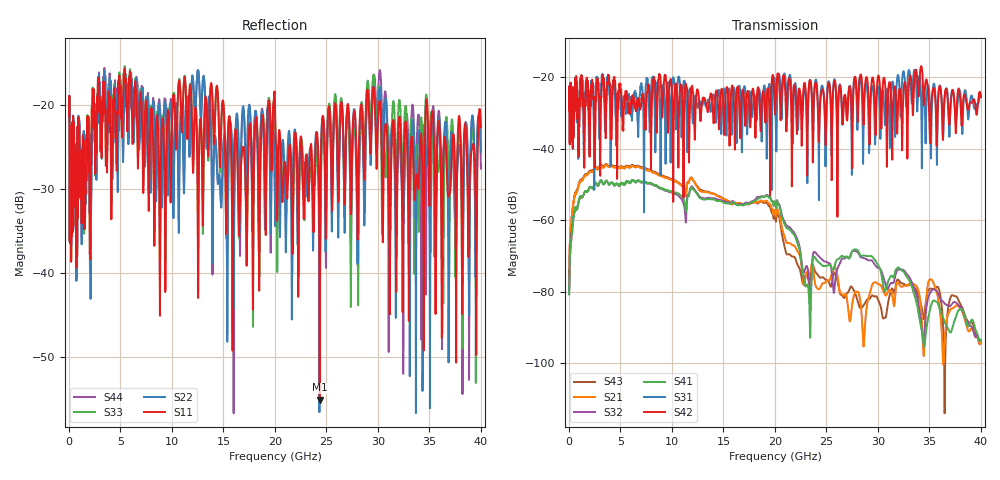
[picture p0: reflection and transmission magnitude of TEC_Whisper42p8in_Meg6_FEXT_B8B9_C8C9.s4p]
! Tyco Electronics Strada Whisper System
! FEXT_B8B9-C8C9
!! SYSTEM DESCRIPTION: Daughtercard-Connector-Backplane-Connector-Daughtercard
!! PCB DESCRIPTION: BP: 250mil, 26 lyrs, Megtron6, bottom layer route, no stub, 6-9-6mil 30" traces; DC: 150mil, 16 lyrs, Megtron6, bottom layer route, no stub, 6-9-6mil 5" traces
!! CONNECTOR DESCRIPTION: STRADA Whisper, Right Angle Receptacle to Vertical Header
!! MODEL DESCRIPTION: Tyco Electronics System 4-port S-parameter
!! MODEL STATUS: Developmental
!! MODEL GEOMETRY: Channel Model
!! MODEL FREQUENCY RANGE: DC to 40 GHz in 10 MHz frequency steps
!! MODEL EDGE RATE LIMITATION: 12.5 ps (Using conservative 0.5/Fmax rule of thumb)
!! TIME-DOMAIN TRANSFORM CAUTIONS:
!! 1.) Do not simulate transient edge rates faster than the number listed above.  Edge rates faster than this number
!!  contain significant spectral content at frequencies above the model's highest frequency.
!! 2.) Even when simulating edge rates that are slower than the number listed above, be aware that the best time
!!  resolution possible with a direct iFFT is (1 / 2Fmax).  As a result, time resolution is typically not adequate
!!  for most time-domain simulations unless tricks such as windowing are used to minimize leakage and aliasing.
!! 3.) Because the model has a uniform frequency step, a direct iFFT will result in an impulse that that has a time
!!  length given by either (1 / Fstep) or (1 / 2Fstep), depending on the transform being used.  Care has been taken
!!  in selecting the frequency step to ensure a settled impulse response for the model.  Therefore, convolution with
!!  the model's impulse response should present no issues.  However, if directly concatenating s-parameter models
!!  in the frequency domain a user must either interpolate necessary interim frequencies or complete impulse response
!!  zero-padding.  Impulse response zero-padding is more difficult, but more accurate.
!! PORT DEFINITIONS:
!! Port  1  ----->  Side A  C8  B8  Side B  <-----  Port  2
!! Port  3  ----->  Side A  C9  B9  Side B  <-----  Port  4
! Created Wed Apr 27 13:57:37 2011
# hz S ma R 50
! 4 Port Network Data from SP1.SP block
! freq  magS11  angS11  magS12  angS12  magS13  angS13  magS14  angS14
!  magS21  angS21  magS22  angS22  magS23  angS23  magS24  angS24
!  magS31  angS31  magS32  angS32  magS33  angS33  magS34  angS34
!  magS41  angS41  magS42  angS42  magS43  angS43  magS44  angS44
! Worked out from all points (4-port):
!   4000 points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, 10 MHz to 40 GHz, reference 50 ohm
!   strongest paths, dB at 10 MHz, 10.01 GHz, 20.01 GHz, 30.01 GHz, 40 GHz:
!     S42: -29.3, -25.0, -30.5, -19.8, -25.6
!     S31: -29.3, -22.6, -23.1, -22.6, -25.3
!     S41: -80.6, -52.0, -55.1, -72.5, -93.4
!     S32: -80.7, -52.3, -54.8, -73.3, -93.4
!     S21: -79.5, -48.8, -57.2, -77.8, -94.3
!     S43: -79.2, -48.6, -58.3, -82.2, -94.1
!   lowest |S11| = -55.1 dB at 24.35 GHz (marker M1), VSWR 1.00, Z = 50 + j0.175 ohm
!   |S11| at or under -10 dB: start of sweep to end of sweep
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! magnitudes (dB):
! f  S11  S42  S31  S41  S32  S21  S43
! 10 MHz  -21.2  -29.3  -29.3  -80.6  -80.7  -79.5  -79.2
! 1.12 GHz  -30.0  -20.8  -20.3  -53.5  -53.6  -49.2  -48.9
! 6.22 GHz  -22.5  -27.0  -27.6  -48.8  -48.9  -44.9  -44.7
! 19.27 GHz  -21.7  -23.4  -29.6  -53.3  -53.0  -54.8  -55.3
! 24.35 GHz  -55.1  -30.0  -29.5  -72.0  -70.3  -79.1  -76.0
! 30.18 GHz  -19.5  -22.1  -30.5  -73.4  -73.5  -77.9  -83.3
! 40 GHz  -22.6  -25.6  -25.3  -93.4  -93.4  -94.3  -94.1
